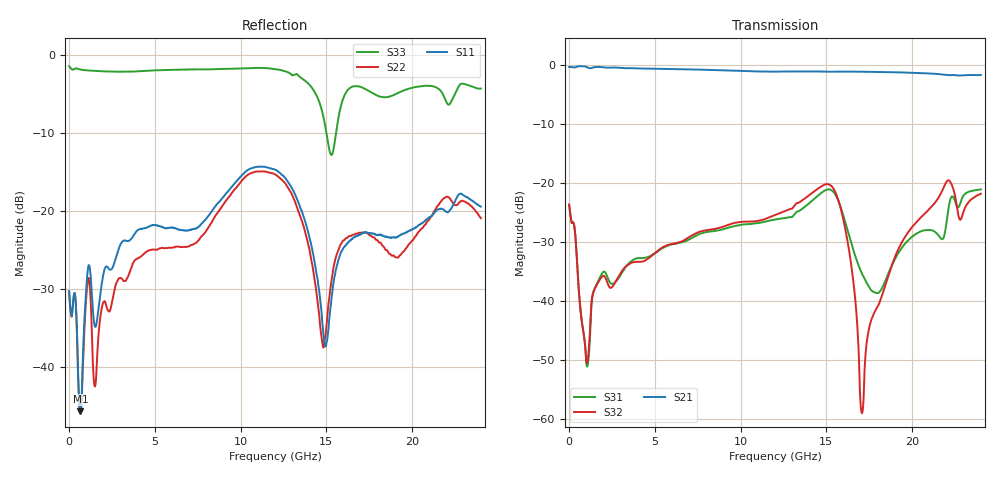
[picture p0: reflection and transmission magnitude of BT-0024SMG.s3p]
! MARKI MICROWAVE INC.
! Email:  info@markimicrowave.com  Phone:  408-778-4200
! Model Number:  BT-0024SM  Date:  12/12
! Filename:		BT_0024SM.S3P  Version: 1.0
! Description:  3-port S-parameter data for Bias Tee BT-0024SM
! Frequency Range: 	10 MHz to 24 GHz
! Port Configuration:	PORT 1: RF & DC
!  PORT 2: RF
!  Port 3: DC
! S3P File: Measurements: Mag<S11> Ang<S11> Mag<S12> Ang<S12> Mag<S13> Ang<S13> ! row 1
!  Mag<S21> Ang<S21> Mag<S22> Ang<S22> Mag<S23> Ang<S23> ! row 2
!  Mag<S31> Ang<S31> Mag<S32> Ang<S32> Mag<S33> Ang<S33> ! row 3
# Hz S  dB  R 50
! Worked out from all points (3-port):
!   801 points, 10 MHz to 24 GHz, reference 50 ohm
!   strongest paths, dB at 10 MHz, 6.008 GHz, 12.01 GHz, 18 GHz, 24 GHz:
!     S21: -0.3, -0.6, -1.0, -1.1, -1.6
!     S32: -23.6, -30.3, -25.4, -40.8, -21.8
!     S31: -23.7, -30.3, -26.1, -38.6, -21.0
!   lowest |S11| = -45.6 dB at 669.7 MHz (marker M1), VSWR 1.01, Z = 50.4 - j0.326 ohm
!   |S11| at or under -10 dB: start of sweep to end of sweep
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1e7  -30.21 145.9  -0.25 -0.9  -23.55 -37.5
     -0.26 -1.1  -30.41 142.8  -23.64 -37.4
     -23.66 -37.2  -23.58 -36.8  -1.37 0.5
6.69725e8  -45.63 -38.2  -0.12 -32.0  -41.49 -102.6
           -0.12 -32.0  -45.91 -33.5  -41.37 -101.1
           -41.49 -102.0  -41.34 -101.0  -1.81 -39.0
3.548525e9  -23.69 71.4  -0.46 -169.0  -33.42 -117.1
            -0.45 -169.2  -27.75 116.3  -33.61 -117.3
            -33.40 -116.7  -33.61 -117.2  -2.08 161.9
7.56685e9  -21.96 -107.8  -0.69 1.1  -28.69 54.2
           -0.70 0.9  -23.67 -65.3  -28.30 58.3
           -28.64 54.1  -28.25 58.5  -1.79 -49.5
9.935862e9  -15.72 158.0  -0.88 -110.5  -27.10 -64.9
            -0.91 -110.9  -16.43 164.0  -26.61 -60.1
            -27.08 -64.9  -26.58 -59.8  -1.68 -174.0
1.2005e10  -14.64 67.7  -1.00 152.7  -26.17 -167.3
           -1.04 152.3  -15.25 62.6  -25.43 -158.4
           -26.13 -167.4  -25.36 -158.4  -1.75 81.4
1.551354e10  -27.95 69.5  -1.00 -12.7  -21.97 -42.4
             -1.05 -13.1  -26.21 90.5  -21.56 -45.3
             -21.86 -42.2  -21.43 -44.9  -10.69 68.4
1.707289e10  -22.85 22.7  -0.99 -86.8  -35.48 -158.1
             -1.06 -87.2  -22.71 7.9  -58.37 -72.4
             -35.31 -158.8  -59.01 -90.3  -4.10 -123.8
2.082132e10  -21.03 -127.5  -1.26 94.3  -27.95 -151.6
             -1.33 94.1  -21.51 172.5  -24.98 -157.4
             -27.92 -152.0  -24.88 -157.3  -3.89 32.9
2.4e10  -19.40 90.8  -1.53 -54.3  -21.12 37.6
        -1.61 -54.4  -20.88 38.8  -21.94 25.9
        -21.03 36.7  -21.76 24.9  -4.25 -135.9
